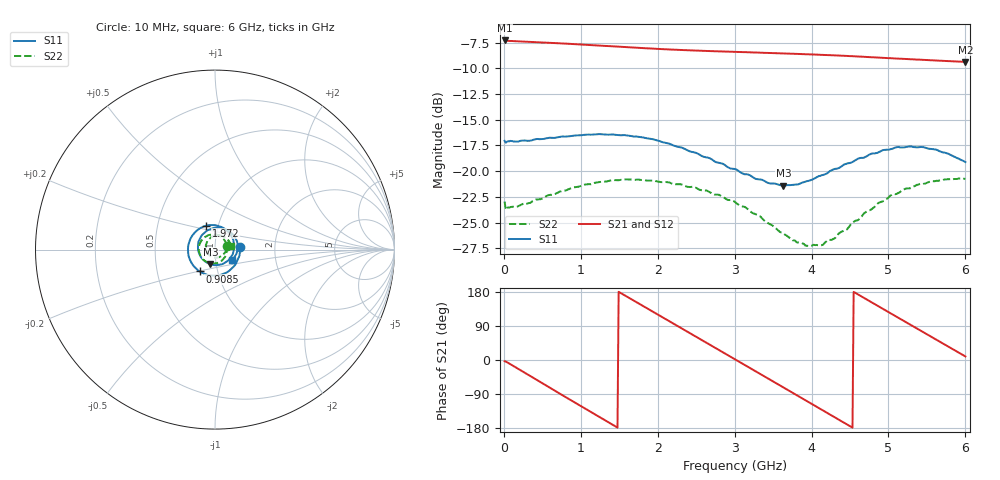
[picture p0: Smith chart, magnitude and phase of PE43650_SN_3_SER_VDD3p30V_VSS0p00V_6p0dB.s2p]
!Keysight Technologies,N5245B,MY57181451,A.13.50.07
!Date: Tuesday, May 07, 2019 07:59:56
!Correction: S11(Full 2 Port(1,2))
!S21(Full 2 Port(1,2))
!S12(Full 2 Port(1,2))
!S22(Full 2 Port(1,2))
!S2P File: Measurements: S11, S21, S12, S22:
# Hz S  dB  R 50
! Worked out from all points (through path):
!   401 points, 10 MHz to 6 GHz, reference 50 ohm
!   highest |S21| = -7.30 dB at 10 MHz (marker M1); lowest = -9.4 dB at 6 GHz (marker M2)
!   group delay of S21, straight-line fit = 328 ps
!   lowest |S11| = -21.4 dB at 3.634 GHz (marker M3), VSWR 1.19, Z = 46.9 - j7.66 ohm
!   |S11| at or under -10 dB: start of sweep to end of sweep
!   |S22| runs from -27.3 to -20.7 dB; largest |S21 - S12| = 0.0033
!   S11 on the Smith chart (normalised r, x): 10 MHz: 1.32, +0.04; 908.5 MHz: 0.82, -0.20; 1.972 GHz: 0.88, +0.24; 6 GHz: 1.20, -0.14
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1e7  -17.06 5.3  -7.30 -3.3  -7.36 -3.2  -22.96 16.8
2.496e8  -17.03 -36.4  -7.41 -31.0  -7.46 -31.0  -23.19 -35.8
5.04175e8  -16.88 -72.0  -7.50 -61.9  -7.55 -61.8  -22.67 -71.9
9.085e8  -16.55 -125.2  -7.65 -110.5  -7.71 -110.5  -21.59 -122.3
1.013325e9  -16.51 -138.5  -7.71 -123.1  -7.75 -123.1  -21.40 -134.6
1.252925e9  -16.41 -167.5  -7.80 -151.6  -7.86 -151.6  -21.06 -160.3
1.47755e9  -16.49 166.0  -7.89 -178.3  -7.96 -178.3  -20.88 176.6
1.71715e9  -16.64 138.4  -8.01 153.3  -8.07 153.3  -20.83 153.1
1.971725e9  -16.98 109.8  -8.11 123.3  -8.16 123.3  -20.97 129.3
2.01665e9  -17.06 104.8  -8.12 118.0  -8.18 118.0  -21.03 125.1
2.241275e9  -17.61 79.3  -8.21 91.6  -8.26 91.6  -21.28 104.0
2.4659e9  -18.16 53.1  -8.28 65.2  -8.33 65.2  -21.56 82.9
2.750425e9  -19.11 19.4  -8.35 31.7  -8.40 31.8  -22.28 55.0
3.005e9  -19.80 -13.7  -8.41 1.8  -8.47 1.9  -23.00 28.6
3.289525e9  -20.78 -53.9  -8.47 -31.8  -8.53 -31.7  -24.24 -5.7
3.63395e9  -21.43 -107.3  -8.56 -72.4  -8.61 -72.3  -26.06 -53.1
4.008325e9  -20.83 -166.0  -8.66 -116.5  -8.71 -116.5  -27.24 -117.2
4.277875e9  -19.85 155.3  -8.74 -148.4  -8.80 -148.4  -26.62 -164.2
4.517475e9  -19.17 123.3  -8.83 -176.8  -8.88 -176.6  -25.12 157.9
5.01165e9  -17.90 65.4  -9.02 125.1  -9.07 125.3  -22.47 97.9
5.4609e9  -17.68 18.6  -9.19 72.4  -9.24 72.6  -21.23 55.1
6e9  -19.13 -31.5  -9.38 9.4  -9.43 9.5  -20.75 11.7
